FUNCTION "SINCRONIZZAZIONE ASSI" : VOID
TITLE =CICLO DI SINCRONIZZAZIONE ASSI
VERSION : 0.1

BEGIN
NETWORK
TITLE =INIZIO SINCRONIZZAZIONE
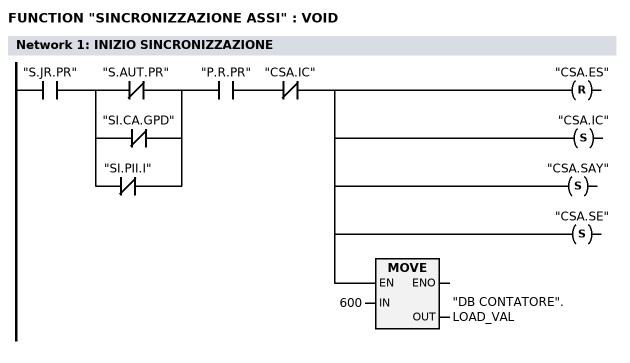
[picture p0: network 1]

      U     "S.JR.PR";
      U(    ;
      ON    "S.AUT.PR";
      ON    "SI.CA.GPD";
      ON    "SI.PII.I";
      )     ;
      U     "P.R.PR";
      UN    "CSA.IC";
      R     "CSA.ES";
      S     "CSA.IC";
      S     "CSA.SAY";
      S     "CSA.SE";

      SPBN  ET01;
      L     600;
      T     "DB CONTATORE".LOAD_VAL;
ET01: NOP   0;

NETWORK
TITLE =SINCRONIZZAZIONE ASSE Y

      U     M    160.1;

      =     L      0.0;
      U     L      0.0;
      U     "CSA.SAY";
      L     S5T#1S500MS;
      SE    "T      14";

      NOP   0;
      NOP   0;
      NOP   0;
      U     "T      14";
      =     M    144.1;
      U     L      0.0;
      U     M    144.1;
      U     "DB ASSE Y".PAST1_11_ImpostPuntoRif;
      FP    "CSA.AAYS";
      S     "CSA.AYS";
      S     "CSA.SAXEZ";
      R     "CSA.SAY";
NETWORK
TITLE =SINCRONIZZAZIONE ASSI X E Z

      U     M    160.1;

      =     L      0.0;
      U     L      0.0;
      U     "CSA.SAXEZ";


      L     S5T#1S500MS;
      SE    "T      31";
      NOP   0;
      NOP   0;
      NOP   0;
      U     "T      31";
      =     M    144.2;
      U     L      0.0;
      U     M    144.2;
      U     "DB ASSE X".PAST1_11_ImpostPuntoRif;
      FP    "CSA.AAXS";
      S     "CSA.AXS";
NETWORK
TITLE =SINCRONIZZAZIONE ASSI X E Z


      U     M    160.1;

      =     L      0.0;
      U     L      0.0;
      U     "CSA.SAXEZ";

      L     S5T#1S500MS;
      SE    "T      43";
      NOP   0;
      NOP   0;
      NOP   0;
      U     "T      43";
      =     M    144.3;
      U     L      0.0;
      U     M    144.3;
      U     "DB ASSE Z".PAST1_11_ImpostPuntoRif;
      FP    "CSA.AAZS";
      S     "CSA.AZS";
NETWORK
TITLE =SINCRONIZZAZIONE ASSI X E Z
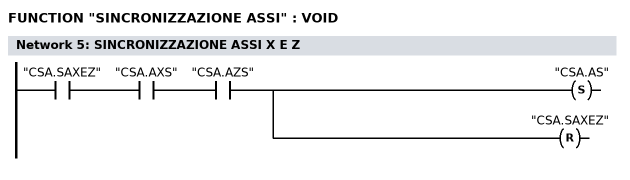
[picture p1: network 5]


      U     "CSA.SAXEZ";
      U     "CSA.AXS";
      U     "CSA.AZS";
      S     "CSA.AS";
      R     "CSA.SAXEZ";

NETWORK
TITLE =SINCRONIZZAZIONE ENCODER

      U     "CSA.SE";
      U     "FP.SI.PCN";
      S     "L_DIRECT";
      S     "CSA.SOE";
      R     "CSA.SE";
//------------------------
      U     "CSA.SOE";
      UN    "L_DIRECT";
      SPBN  ET02;
      L     2047;
      T     "DB CONTATORE".LOAD_VAL;
      S     "L_PREPAR";
ET02: NOP   0;
//------------------------
      U     "CSA.SOE";
      UN    "L_DIRECT";
      U(    ;
      L     "DB CONTATORE".ACT_LOAD;
      L     1500;
      >=D   ;
      )     ;
      S     "CSA.ES";
      R     "CSA.SOE";

NETWORK
TITLE =CONCLUSIONE CICLO SINCRONIZZAZIONE
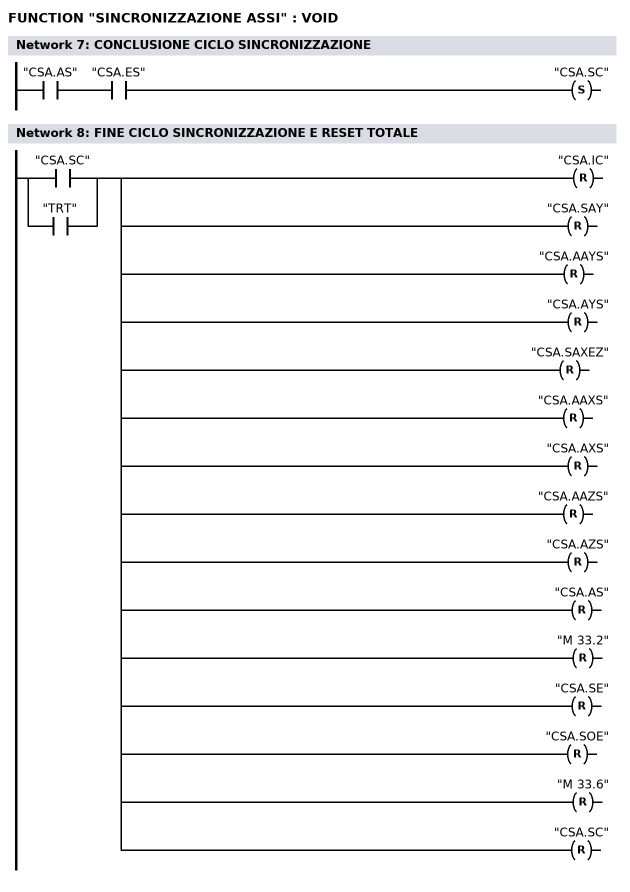
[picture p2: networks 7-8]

      U     "CSA.AS";
      U     "CSA.ES";
      S     "CSA.SC";

NETWORK
TITLE =FINE CICLO SINCRONIZZAZIONE E RESET TOTALE

      O     "CSA.SC";
      O     "TRT";
      R     "CSA.IC";
      R     "CSA.SAY";
      R     "CSA.AAYS";
      R     "CSA.AYS";
      R     "CSA.SAXEZ";
      R     "CSA.AAXS";
      R     "CSA.AXS";
      R     "CSA.AAZS";
      R     "CSA.AZS";
      R     "CSA.AS";
      R     "M      33.2";
      R     "CSA.SE";
      R     "CSA.SOE";
//      R     "CSA.ES"
      R     "M      33.6";
      R     "CSA.SC";



END_FUNCTION

